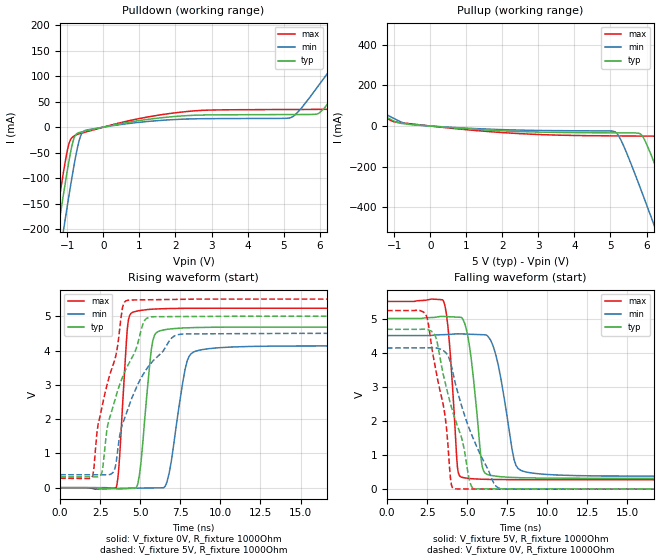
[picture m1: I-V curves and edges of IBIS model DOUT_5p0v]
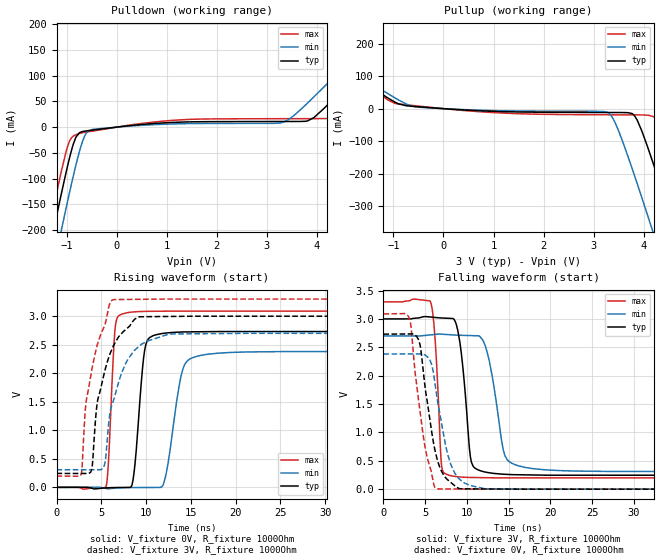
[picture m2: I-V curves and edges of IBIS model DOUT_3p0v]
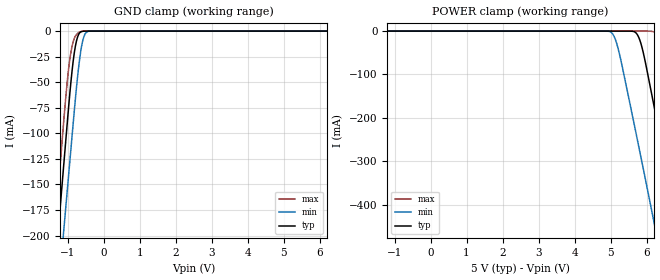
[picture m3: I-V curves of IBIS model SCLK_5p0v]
|Texas Instruments Incorporated
| DAC088S085: 8-Bit Micro Power OCTAL Digital-to-Analog Converter with
|Rail-to-Rail Outputs
| Marketing part#   Digital Voltage Range   Package-type   #pins
| DAC088S085CISQ   2.7 to 5.5 V   LLP   16
| DAC088S085CIMT   2.7 to 5.5 V   TSSOP   16
[IBIS Ver]   4.0
[File name]   dac088s085.ibs
[File Rev]   1.0
[Date]   01/19/2012
[Source]   Texas Instruments Incorporated.
   Analog-eLab, HPA
   12500 TI Blvd
   Dallas, TX -75243
   For Support e-mail: elab_ibis@list.ti.com
[Notes]   Revision History:
   1.0: 01/19/2012
   - Initial version of the model
   - Initial Model generated from simulations
   - Model not matched to measurements
   - Models with trailing _5p0v are generated based on 5.0V
   power supply.
   - Models with trailing _3p0v are generated based on 3.0V
   power supply.
   - C_comp although listed in numerical order of value are
   obtained from varying PVT conditions. For PVT conditions
   for each specific value refer the buffer description under
   respective [Model]. IBIS model user is responsible for using
   appropriate C_comp to simulate for Signal Integrity.
[Disclaimer]
  This model is designed as an aid for customers of Texas Instruments.
  TI and its licensors and suppliers make no warranties, either expressed
  or implied, with respect to this model, including the warranties of
  merchantability or fitness for a particular purpose.  The model is
  provided solely on an "as is" basis.  The entire risk as to its quality
  and performance is with the customer.
[Copyright] (C) Copyright 2012 Texas Instruments Incorporated.
   All rights reserved.
|   Device
[Component]   DAC088S085CISQ
[Manufacturer] TI
[Package]   | 16 pin LLP
| variable   typ   min   max
R_pkg   0.01   0.008   0.12
L_pkg   0.1nH   0.08nH   0.12nH
C_pkg   0.1pF   0.08pF   0.12pF
|-------------------------PIN------------------------------------------------
[Pin] signal_name  model_name  R_pin  L_pin C_pin
1   VOUTA   TERM   NA   NA   NA
2   VOUTB   TERM   NA   NA   NA
3   VOUTC   TERM   NA   NA   NA
4   VOUTD   TERM   NA   NA   NA
5   VA   POWER   NA   NA   NA
6   VREF1   TERM   NA   NA   NA
7   VREF2   TERM   NA   NA   NA
8   GND   GND   NA   NA   NA
9   VOUTH   TERM   NA   NA   NA
10   VOUTG   TERM   NA   NA   NA
11   VOUTF   TERM   NA   NA   NA
12   VOUTE   TERM   NA   NA   NA
13   SYNCB   SYNCB   NA   NA   NA
14   SCLK   SCLK   NA   NA   NA
15   DIN   SCLK   NA   NA   NA
16   DOUT   DOUT   NA   NA   NA
17   PAD   GND   NA   NA   NA
[Component]   DAC088S085CIMT
[Manufacturer] TI
[Package]   | 16 pin TSSOP
| variable   typ   min   max
R_pkg   0.01   0.008   0.12
L_pkg   0.1nH   0.08nH   0.12nH
C_pkg   0.1pF   0.08pF   0.12pF
|-------------------------PIN------------------------------------------------
[Pin] signal_name  model_name  R_pin  L_pin C_pin
1   DIN   SCLK   NA   NA   NA
2   DOUT   DOUT   NA   NA   NA
3   VOUTA   TERM   NA   NA   NA
4   VOUTB   TERM   NA   NA   NA
5   VOUTC   TERM   NA   NA   NA
6   VOUTD   TERM   NA   NA   NA
7   VA   POWER   NA   NA   NA
8   VREF1   TERM   NA   NA   NA
9   VREF2   TERM   NA   NA   NA
10   GND   GND   NA   NA   NA
11   VOUTH   TERM   NA   NA   NA
12   VOUTG   TERM   NA   NA   NA
13   VOUTF   TERM   NA   NA   NA
14   VOUTE   TERM   NA   NA   NA
15   SYNCB   SYNCB   NA   NA   NA
16   SCLK   SCLK   NA   NA   NA
[Model Selector] DOUT
DOUT_5p0v   model for 5.0v operation
DOUT_3p0v   model for 3.0v operation
[Model Selector] SCLK
SCLK_5p0v   model for 5.0v operation
SCLK_3p0v   model for 3.0v operation
[Model Selector] SYNCB
SYNCB_5p0v   model for 5.0v operation
SYNCB_3p0v   model for 3.0v operation
[Model Selector] TERM
TERM_5p0v   model for 5.0v operation
TERM_3p0v   model for 3.0v operation
|   Model
[Model] TERM_5p0v
Model_type Terminator
C_comp   1fF   1fF   1fF
| variable   typ   min   max
[Voltage Range]   5.0V   4.5V   5.5V
[POWER Clamp Reference]  3.3V   3.0V   3.6V
[GND Clamp Reference]   0.0V   0.0V   0.0V
|Operating Temperature
[Temperature Range]   27   85   -40
|   Model
[Model] TERM_3p0v
Model_type Terminator
C_comp   1fF   1fF   1fF
| variable   typ   min   max
[Voltage Range]   3.0V   2.7V   3.3V
[POWER Clamp Reference]  3.3V   3.0V   3.6V
[GND Clamp Reference]   0.0V   0.0V   0.0V
|Operating Temperature
[Temperature Range]   27   85   -40
| Models and submodels in the file (8): DOUT_5p0v (Output), DOUT_3p0v (Output), SCLK_5p0v (Input), SCLK_3p0v (Input), SYNCB_5p0v (Input), SYNCB_3p0v (Input), TERM_5p0v (Terminator), TERM_3p0v (Terminator)
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|   Model
[Model]   DOUT_5p0v
Model_type   Output
Polarity   Non-Inverting
Vmeas = 2.5
Vref = 2.5
Cref = 1pF
Rref = 1000000
|   typ   min   max
C_comp   0.916pF   0.856pF   0.959pF
[Voltage Range]   5   4.5   5.5
[Temperature Range]   27   125   -40
[Pullup Reference]   5   4.5   5.5
[Pulldown Reference]   0   0   0
[Power Clamp Reference]   5   4.5   5.5
[GND Clamp Reference]   0   0   0
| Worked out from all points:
|   slope of the pulldown table from 0 to 0.75 V, typ, clamps not added: 73.7 ohm
|   slope of the pullup table from 0 to 0.75 V, typ, clamps not added: 71.2 ohm
|   falling waveform, V_fixture 5V, R_fixture 1000Ohm: 20-80 % time 608ps typ, 870ps min, 438ps max; typ from 5 V to 0.317 V
|   rising waveform, V_fixture 0V, R_fixture 1000Ohm: 20-80 % time 541ps typ, 786ps min, 394ps max; typ from 0 V to 4.68 V
|   rising waveform, V_fixture 5V, R_fixture 1000Ohm: 20-80 % time 1.94ns typ, 2.14ns min, 1.43ns max; typ from 0.317 V to 5 V
|   falling waveform, V_fixture 0V, R_fixture 1000Ohm: 20-80 % time 1.54ns typ, 1.86ns min, 1.06ns max; typ from 4.68 V to 0 V
[Pulldown]
|   Voltage   I(typ)   I(min)   I(max)
-5V       -2.033A    -2.097A    -1.993A
-1.385V   -260.3mA   -332.1mA   -215.2mA
-1.235V   -189.8mA   -261.4mA   -145mA
-1.115V   -134.9mA   -205.8mA   -91.14mA
-965mV    -70.17mA   -138.2mA   -34.83mA
-815mV    -21.53mA   -74.94mA   -17.43mA
-515mV    -7.89mA    -6.741mA   -10.02mA
5.185V    24.64mA    18.36mA    34.56mA
5.995V    27.9mA     84.03mA    34.82mA
6.625V    85.88mA    144.5mA    36.6mA
7.105V    135.1mA    190.7mA    85.06mA
9.985V    430.4mA    467.3mA    429mA
[Pullup]
|   Voltage   I(typ)   I(min)   I(max)
-5V       431mA      419.8mA    489.5mA
-1.025V   25.7mA     38.54mA    21.89mA
235mV     -3.501mA   -2.707mA   -4.612mA
5.125V    -33.69mA   -28.62mA   -48.75mA
5.335V    -33.86mA   -86.09mA   -49.01mA
5.845V    -41.28mA   -313.9mA   -49.54mA
6.265V    -205.2mA   -514.7mA   -50.06mA
6.535V    -332.8mA   -645.5mA   -68.62mA
6.895V    -506.6mA   -821.2mA   -221.6mA
7.195V    -653.1mA   -968.1mA   -365.2mA
7.615V    -859.3mA   -1.174A    -569.9mA
9.985V    -2.026A    -2.334A    -1.739A
[Ramp]
R_load = 1000
|   typ   min   max
dV/dt_r   2.80983/5.40792e-10   2.48125/7.85781e-10   3.1396/3.94024e-10
dV/dt_f   2.80967/6.07821e-10   2.47319/8.70189e-10   3.13532/4.37912e-10
[Falling Waveform]
V_fixture = 5V
V_fixture_min = 4.5V
V_fixture_max = 5.5V
R_fixture = 1000Ohm
C_fixture = 0F
|   Time   V(typ)   V(min)   V(max)
0s        5V         4.5V       5.5V
3.506ns   5.061V     4.527V     5.528V
3.892ns   5.052V     4.535V     4.294V
4.401ns   5.039V     4.551V     612.6mV
5.074ns   4.394V     4.541V     315.1mV
5.952ns   642.3mV    4.525V     290.5mV
7.061ns   365.6mV    3.344V     281.7mV
8.056ns   340.3mV    689.5mV    279mV
9.861ns   324mV      433.9mV    275.1mV
100ns     317.2mV    378mV      274.5mV
[Rising Waveform]
V_fixture = 0V
V_fixture_min = 0V
V_fixture_max = 0V
R_fixture = 1000Ohm
C_fixture = 0F
|   Time   V(typ)   V(min)   V(max)
0s        10.55uV    612.7nV    -29.84uV
3.506ns   -22.73mV   -27.63mV   14.77mV
4.272ns   -10.4mV    -24.72mV   4.913V
4.846ns   113.1mV    -13.84mV   5.156V
5.433ns   2.818V     -9.202mV   5.194V
6.032ns   4.529V     -5.774mV   5.212V
6.809ns   4.625V     435.8mV    5.223V
7.93ns    4.661V     3.703V     5.229V
9.861ns   4.679V     4.079V     5.232V
100ns     4.683V     4.135V     5.233V
[Rising Waveform]
V_fixture = 5V
V_fixture_min = 4.5V
V_fixture_max = 5.5V
R_fixture = 1000Ohm
C_fixture = 0F
|   Time   V(typ)   V(min)   V(max)
0s        317.2mV    378mV      274.4mV
2.04ns    313.2mV    376.4mV    356.1mV
2.616ns   461.1mV    376mV      2.363V
2.983ns   1.859V     375.7mV    3.102V
3.352ns   2.452V     481.9mV    3.648V
3.892ns   3.226V     1.855V     5.252V
4.272ns   3.606V     2.351V     5.469V
5.383ns   4.937V     3.451V     5.479V
7.637ns   4.99V      4.48V      5.493V
100ns     5V         4.5V       5.5V
[Falling Waveform]
|Gnd
V_fixture = 0V
V_fixture_min = 0V
V_fixture_max = 0V
R_fixture = 1000Ohm
C_fixture = 0F
|   Time   V(typ)   V(min)   V(max)
0s        4.683V     4.135V     5.233V
2.457ns   4.685V     4.141V     5.078V
3.055ns   4.434V     4.138V     3.469V
3.636ns   3.11V      4.012V     2.094V
4.022ns   2.399V     3.597V     118.9mV
4.228ns   2.083V     3.174V     9.5mV
5.267ns   82.66mV    1.612V     6.144mV
6.66ns    7.504mV    178.8mV    4.191mV
7.324ns   7.45mV     6.922mV    3.261mV
100ns     18.46uV    12.84uV    -18.18uV
|   Model
[Model]   DOUT_3p0v
Model_type   Output
Polarity   Non-Inverting
Vmeas = 1.5
Vref = 1.5
Cref = 1pF
Rref = 1000000
|   typ   min   max
C_comp   0.916pF   0.856pF   0.959pF
[Voltage Range]   3   2.7   3.3
[Temperature Range]   27   125   -40
[Pullup Reference]   3   2.7   3.3
[Pulldown Reference]   0   0   0
[Power Clamp Reference]   3   2.7   3.3
[GND Clamp Reference]   0   0   0
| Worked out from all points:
|   slope of the pulldown table from 0 to 0.45 V, typ, clamps not added: 95.2 ohm
|   slope of the pullup table from 0 to 0.45 V, typ, clamps not added: 103 ohm
|   falling waveform, V_fixture 3V, R_fixture 1000Ohm: 20-80 % time 977ps typ, 1.51ns min, 623ps max; typ from 3 V to 0.244 V
|   rising waveform, V_fixture 0V, R_fixture 1000Ohm: 20-80 % time 825ps typ, 1.33ns min, 540ps max; typ from 0 V to 2.73 V
|   rising waveform, V_fixture 3V, R_fixture 1000Ohm: 20-80 % time 2.09ns typ, 2.25ns min, 1.93ns max; typ from 0.244 V to 3 V
|   falling waveform, V_fixture 0V, R_fixture 1000Ohm: 20-80 % time 1.71ns typ, 1.85ns min, 1.61ns max; typ from 2.73 V to 0 V
[Pulldown]
|   Voltage   I(typ)   I(min)   I(max)
-3V       -1.048A    -1.117A    -1.006A
-1.353V   -245mA     -316.9mA   -199.9mA
-1.101V   -128.3mA   -199.3mA   -84.65mA
-939mV    -59.33mA   -126.6mA   -26.84mA
-741mV    -10.86mA   -46.85mA   -12.24mA
-615mV    -7.462mA   -13.3mA    -9.803mA
-453mV    -5.458mA   -4.123mA   -7.288mA
3.291V    11.01mA    8.558mA    16.44mA
3.813V    12.1mA     46.77mA    16.54mA
4.227V    44.56mA    86.37mA    16.91mA
4.677V    90.4mA     129.6mA    56.95mA
5.991V    225.1mA    255.8mA    213.7mA
[Pullup]
|   Voltage   I(typ)   I(min)   I(max)
-3V       225.8mA    227.5mA    250.4mA
-975mV    20.56mA    33.66mA    16.44mA
-489mV    5.631mA    4.415mA    7.698mA
3.291V    -11.87mA   -12.79mA   -18.93mA
3.471V    -11.94mA   -58.41mA   -19.04mA
3.813V    -21.3mA    -205mA     -19.23mA
4.191V    -169.5mA   -382.6mA   -24.44mA
4.299V    -219.7mA   -434.3mA   -45.82mA
4.551V    -339.6mA   -555.9mA   -152.5mA
4.947V    -531.5mA   -748.6mA   -341mA
5.289V    -698.7mA   -915.9mA   -507.6mA
5.991V    -1.044A    -1.26A     -853mA
[Ramp]
R_load = 1000
|   typ   min   max
dV/dt_r   1.63883/8.25165e-10   1.42868/1.33452e-09   1.85308/5.39752e-10
dV/dt_f   1.65364/9.76659e-10   1.43449/1.50631e-09   1.86159/6.23404e-10
[Falling Waveform]
V_fixture = 3V
V_fixture_min = 2.7V
V_fixture_max = 3.3V
R_fixture = 1000Ohm
C_fixture = 0F
|   Time   V(typ)   V(min)   V(max)
0s        3V         2.7V       3.3V
5.656ns   3.033V     2.719V     3.298V
6.988ns   3.016V     2.731V     394.3mV
7.899ns   3.01V      2.722V     243.3mV
9.147ns   2.603V     2.712V     215.3mV
10.56ns   471.5mV    2.706V     205.9mV
12.2ns    300.8mV    2.525V     202.3mV
14.57ns   262.2mV    588.1mV    198.4mV
16.93ns   252.5mV    384.2mV    198.4mV
100ns     243.9mV    309.2mV    197.3mV
[Rising Waveform]
V_fixture = 0V
V_fixture_min = 0V
V_fixture_max = 0V
R_fixture = 1000Ohm
C_fixture = 0F
|   Time   V(typ)   V(min)   V(max)
0s        1.869uV    3.33uV     594.7nV
5.565ns   -8.452mV   -19.74mV   28.75mV
6.602ns   -3.534mV   -13.57mV   2.861V
7.899ns   -2.142mV   -4.047mV   3.061V
8.65ns    249.4mV    -3.66mV    3.075V
9.974ns   2.503V     -2.987mV   3.085V
11.67ns   2.693V     696.1uV    3.087V
14.14ns   2.724V     2.09V      3.088V
16.2ns    2.727V     2.316V     3.088V
100ns     2.731V     2.381V     3.088V
[Rising Waveform]
V_fixture = 3V
V_fixture_min = 2.7V
V_fixture_max = 3.3V
R_fixture = 1000Ohm
C_fixture = 0F
|   Time   V(typ)   V(min)   V(max)
0s        243.9mV    309.2mV    197.3mV
2.759ns   242.8mV    308.8mV    236.7mV
3.27ns    242.6mV    308.8mV    1.456V
3.816ns   266.7mV    308.7mV    1.949V
4.525ns   1.461V     308.6mV    2.482V
5.334ns   2.005V     380.9mV    2.821V
6.345ns   2.478V     1.519V     3.289V
8.698ns   2.941V     2.4V       3.295V
12.71ns   2.995V     2.688V     3.3V
100ns     3V         2.7V       3.3V
[Falling Waveform]
|Gnd
V_fixture = 0V
V_fixture_min = 0V
V_fixture_max = 0V
R_fixture = 1000Ohm
C_fixture = 0F
|   Time   V(typ)   V(min)   V(max)
0s        2.731V     2.381V     3.088V
3.136ns   2.735V     2.383V     2.998V
4.402ns   2.534V     2.384V     1.355V
5.074ns   1.709V     2.358V     678.7mV
5.735ns   1.061V     2.218V     308.4mV
6.345ns   584.1mV    1.692V     6.903mV
7.563ns   184.2mV    703.5mV    3.726mV
8.512ns   64.52mV    295mV      3.09mV
12.24ns   3.797mV    7.965mV    594.9uV
100ns     12.43uV    22.03uV    6.18uV
|   Model
[Model]   SCLK_5p0v
Model_type   Input
Vinl = 0.8
Vinh = 2.4
|   typ   min   max
C_comp   0.662pF   0.641pF   0.770pF
[Voltage Range]   5   4.5   5.5
[Temperature Range]   27   125   -40
[Power Clamp Reference]   5   4.5   5.5
[GND Clamp Reference]   0   0   0
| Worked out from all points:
|   GND clamp passes 1 mA (typ) near -0.64 V on its own axis
[GND Clamp]
|   Voltage   I(typ)   I(min)   I(max)
-5V       -1.813A    -1.827A    -1.812A
-1.355V   -235.3mA   -295.2mA   -195.6mA
-1.325V   -222.5mA   -282.9mA   -182.5mA
-1.235V   -184.3mA   -246.3mA   -143.1mA
-1.115V   -133.7mA   -197.8mA   -90.75mA
-995mV    -83.26mA   -149.6mA   -43.85mA
-905mV    -48.31mA   -113.7mA   -19.81mA
-785mV    -14.76mA   -66.35mA   -4.887mA
-635mV    -791uA     -19.45mA   -496.3uA
-515mV    -40.35uA   -2.742mA   -21.44uA
-365mV    -522.8nA   -51.88uA   0A
9.985V    0A         0A         0A
[POWER Clamp]
|   Voltage   I(typ)   I(min)   I(max)
-5V       0A         0A         0A
5.005V    0A         -2.188mA   0A
5.095V    0A         -11.61mA   0A
5.215V    0A         -41.65mA   0A
5.755V    -9.682mA   -254.4mA   0A
5.905V    -48.32mA   -315.6mA   -469.1nA
6.205V    -171.6mA   -439.3mA   -1.751mA
6.265V    -197mA     -464.2mA   -3.842mA
6.475V    -286.4mA   -551.6mA   -37.4mA
6.865V    -453.8mA   -714.9mA   -200mA
7.495V    -725.9mA   -979.8mA   -477.9mA
9.985V    -1.807A    -2.032A    -1.583A
